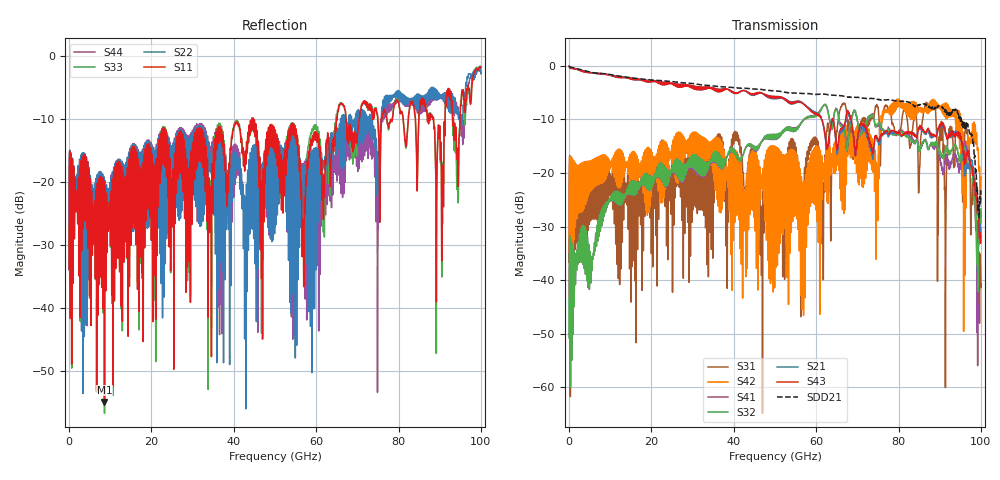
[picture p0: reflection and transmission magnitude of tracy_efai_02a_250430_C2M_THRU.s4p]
!! PART DESCRIPTION: TE 224G+ VSR Channel- Chip to module, IO connector to CPC(Co-packaged connector) through over the board cable
!! CHANNEL DESCRIPTION: Module trace -> Mated IO 224G+ Connector -> Internal Cable Termination -> 30AWG 300mm Cable -> Cable
!!  termination + CPC connector(No footprint or package included)
!! MODEL REVISION:  Rev 3, Created on April 29, 2025
!! MODEL STATUS: Development
!! MODEL GEOMETRY: THRU
!! MODEL FREQUENCY RANGE: 0 GHz to 100 GHz in 10.00 MHz frequency steps
!! PORT DEFINITIONS:
!! Port  1  ----->  Module Side  -->  Host Side  <-----  Port  2
!! Port  3  ----->  Module Side  -->  Host Side  <-----  Port  4
# HZ S MA R 45.000000
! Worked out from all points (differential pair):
!   10000 points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, 10 MHz to 100 GHz, reference 45 ohm
!   strongest paths, dB at 10 MHz, 25.01 GHz, 50.01 GHz, 75.01 GHz, 100 GHz:
!     S43: -0.1, -3.3, -5.9, -13.7, -31.8
!     S21: -0.1, -3.3, -6.1, -13.8, -30.2
!     S32: -50.7, -19.8, -12.8, -10.9, -26.7
!     S41: -50.7, -20.0, -12.9, -11.2, -27.4
!     S42: -36.7, -15.4, -16.5, -24.1, -20.8
!     S31: -36.5, -17.8, -16.0, -7.7, -40.6
!   taken as a pair (ports 3,1 in; 4,2 out), SDD21 dB: 0.0, -2.9, -4.7, -6.3, -23.2
!   lowest |S11| = -54.9 dB at 8.6 GHz (marker M1), VSWR 1.00, Z = 44.9 + j0.15 ohm
!   |S11| at or under -10 dB: start of sweep to 44.32 GHz; 44.72 GHz to 64.9 GHz (20.18 GHz wide, 36.8 % of centre); 67.23 GHz to 70.41 GHz (3.185 GHz wide, 4.63 % of centre)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
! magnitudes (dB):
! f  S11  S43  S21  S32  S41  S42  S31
! 10 MHz  -33.8  -0.1  -0.1  -50.7  -50.7  -36.7  -36.5
! 8.6 GHz  -54.9  -1.5  -1.5  -26.8  -26.9  -21.5  -27.5
! 56.35 GHz  -20.4  -6.8  -6.8  -10.6  -10.6  -22.5  -31.4
! 66.47 GHz  -7.6  -11.5  -12.2  -11.6  -11.0  -14.2  -7.2
! 88.17 GHz  -9.4  -12.7  -13.2  -14.2  -14.7  -7.5  -7.5
! 96.6 GHz  -5.1  -16.8  -19.1  -18.5  -15.9  -15.1  -12.2
! 100 GHz  -1.8  -31.8  -30.2  -26.7  -27.4  -20.8  -40.6
